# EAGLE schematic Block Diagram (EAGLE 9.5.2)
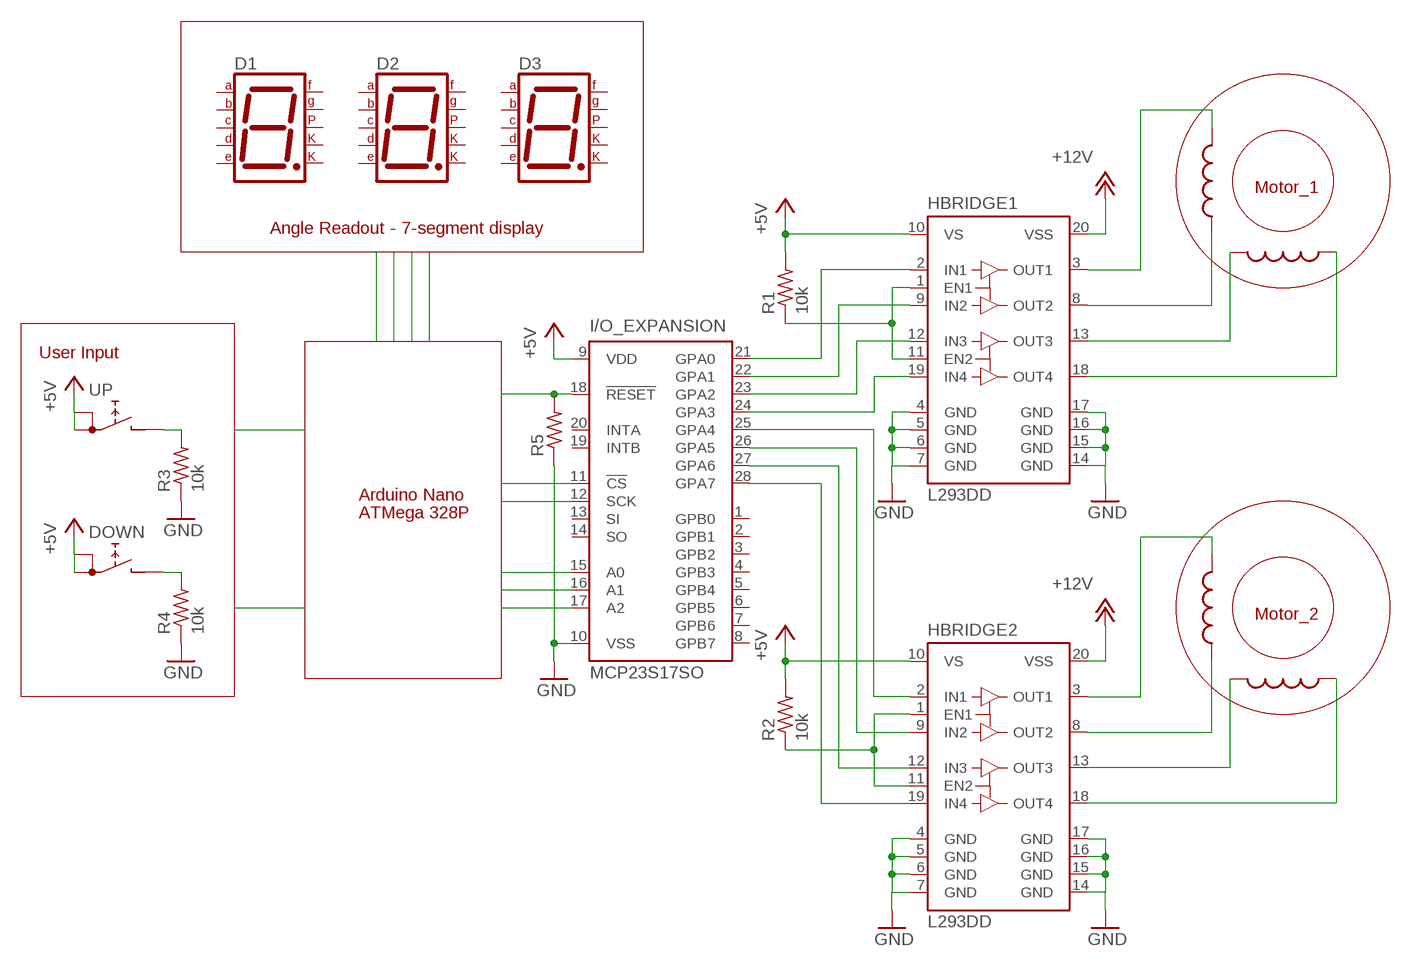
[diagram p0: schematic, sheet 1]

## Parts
D1  7SEG-MCK  [7SEG-7]
D2  7SEG-MCK  [7SEG-7]
D3  7SEG-MCK  [7SEG-7]
DOWN  RDT1034  [RDT1034]
HBRIDGE1  L293DD  [SO20]
HBRIDGE2  L293DD  [SO20]
I/O_EXPANSION  MCP23S17SO  [SO28W]
L1  L-US0207/15  [0207/15]
L2  L-US0207/15  [0207/15]
L3  L-US0207/15  [0207/15]
L4  L-US0207/15  [0207/15]
R1  10k  R-US_R0805  [R0805]
R2  10k  R-US_R0805  [R0805]
R3  10k  R-US_R0805  [R0805]
R4  10k  R-US_R0805  [R0805]
R5  10k  R-US_R0805  [R0805]
UP  RDT1034  [RDT1034]

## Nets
+5V: HBRIDGE1.10(VS) HBRIDGE2.10(VS) I/O_EXPANSION.9(VDD) R1.2 R2.2
+12V: HBRIDGE1.20(VSS) HBRIDGE2.20(VSS)
GND: HBRIDGE1.4(GND) HBRIDGE1.5(GND) HBRIDGE1.6(GND) HBRIDGE1.7(GND) HBRIDGE1.14(GND) HBRIDGE1.15(GND) HBRIDGE1.16(GND) HBRIDGE1.17(GND) HBRIDGE2.4(GND) HBRIDGE2.5(GND) HBRIDGE2.6(GND) HBRIDGE2.7(GND) HBRIDGE2.14(GND) HBRIDGE2.15(GND) HBRIDGE2.16(GND) HBRIDGE2.17(GND) I/O_EXPANSION.10(VSS) R3.1 R4.1 R5.1
N$1: HBRIDGE1.3(OUT1) L1.2
N$2: HBRIDGE1.8(OUT2) L1.1
N$3: HBRIDGE1.13(OUT3) L2.2
N$4: HBRIDGE1.18(OUT4) L2.1
N$5: HBRIDGE2.3(OUT1) L3.2
N$6: HBRIDGE2.8(OUT2) L3.1
N$7: HBRIDGE1.1(EN1) HBRIDGE1.11(EN2) R1.1
N$8: HBRIDGE2.13(OUT3) L4.2
N$9: HBRIDGE2.18(OUT4) L4.1
N$10: HBRIDGE2.1(EN1) HBRIDGE2.11(EN2) R2.1
N$11: DOWN.B R4.2
N$12: R3.2 UP.B
N$13: UP.A UP.A1 ; supply symbol labelled +5V
N$14: DOWN.A DOWN.A1 ; supply symbol labelled +5V
N$21: HBRIDGE1.2(IN1) I/O_EXPANSION.21(GPA0)
N$22: HBRIDGE1.9(IN2) I/O_EXPANSION.22(GPA1)
N$23: I/O_EXPANSION.11(!CS)
N$24: I/O_EXPANSION.12(SCK)
N$25: I/O_EXPANSION.15(A0)
N$26: I/O_EXPANSION.16(A1)
N$27: I/O_EXPANSION.17(A2)
N$28: I/O_EXPANSION.18(!RESET) R5.2
N$29: HBRIDGE1.12(IN3) I/O_EXPANSION.23(GPA2)
N$30: HBRIDGE1.19(IN4) I/O_EXPANSION.24(GPA3)
N$31: HBRIDGE2.2(IN1) I/O_EXPANSION.25(GPA4)
N$32: HBRIDGE2.9(IN2) I/O_EXPANSION.26(GPA5)
N$33: HBRIDGE2.12(IN3) I/O_EXPANSION.27(GPA6)
N$34: HBRIDGE2.19(IN4) I/O_EXPANSION.28(GPA7)
Unconnected: D1.1(CK1) D1.2(F) D1.3(G) D1.4(E) D1.5(D) D1.6(CK2) D1.7(DP) D1.8(C) D1.9(B) D1.10(A) D2.1(CK1) D2.2(F) D2.3(G) D2.4(E) D2.5(D) D2.6(CK2) D2.7(DP) D2.8(C) D2.9(B) D2.10(A) D3.1(CK1) D3.2(F) D3.3(G) D3.4(E) D3.5(D) D3.6(CK2) D3.7(DP) D3.8(C) D3.9(B) D3.10(A) I/O_EXPANSION.1(GPB0) I/O_EXPANSION.2(GPB1) I/O_EXPANSION.3(GPB2) I/O_EXPANSION.4(GPB3) I/O_EXPANSION.5(GPB4) I/O_EXPANSION.6(GPB5) I/O_EXPANSION.7(GPB6) I/O_EXPANSION.8(GPB7) I/O_EXPANSION.13(SI) I/O_EXPANSION.14(SO) I/O_EXPANSION.19(INTB) I/O_EXPANSION.20(INTA)

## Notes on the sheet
- Motor_1
- Angle Readout - 7-segment display
- User Input
- Arduino Nano
- ATMega 328P
- Motor_2

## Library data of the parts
D1-D3 = special:7SEG-MCK: 7-segment DISPLAY single cathode, 13 mm
DOWN UP = switch:RDT1034: PUSH SWITCH www.radiohm.com
HBRIDGE1 HBRIDGE2 = st-microelectronics:L293DD: PUSH-PULL FOUR CHANNEL DRIVER WITH DIODES Source: http://www.st.com/stonline/books/pdf/docs/1330.pdf; OC_FARNELL: unknown
I/O_EXPANSION = microchip:MCP23S17: http://ww1.microchip.com/downloads/en/DeviceDoc/21952a.pdf Source: http://ww1.microchip.com/downloads/en/DeviceDoc/21952a.pdf; MF: MICROCHIP; MPN: MCP23S17-E/SO; OC_FARNELL: unknown; OC_NEWARK: 31K2950
L1-L4 = rcl:L-US: INDUCTOR, American symbol; SPICEPREFIX: L
R1-R5 = rcl:R-US_: RESISTOR, American symbol; SPICEPREFIX: R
